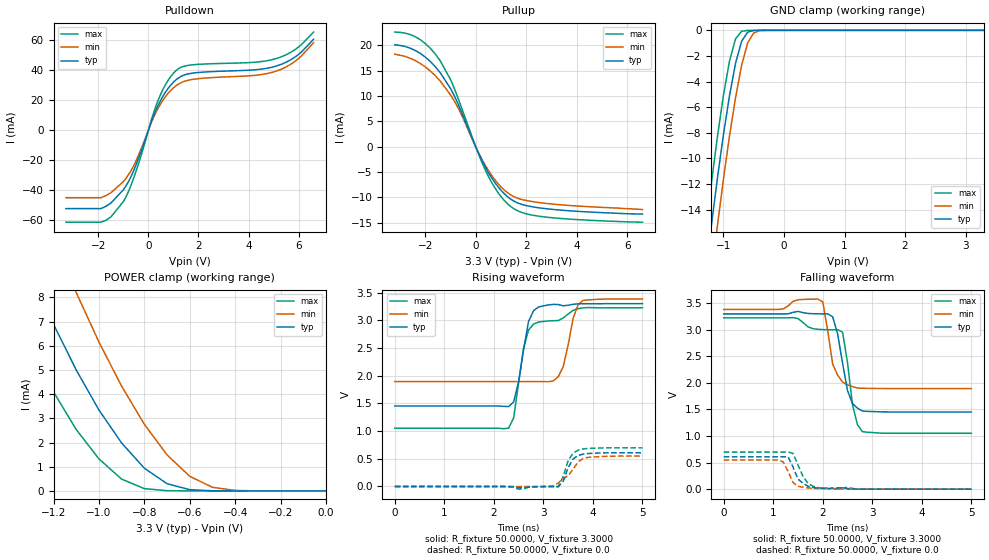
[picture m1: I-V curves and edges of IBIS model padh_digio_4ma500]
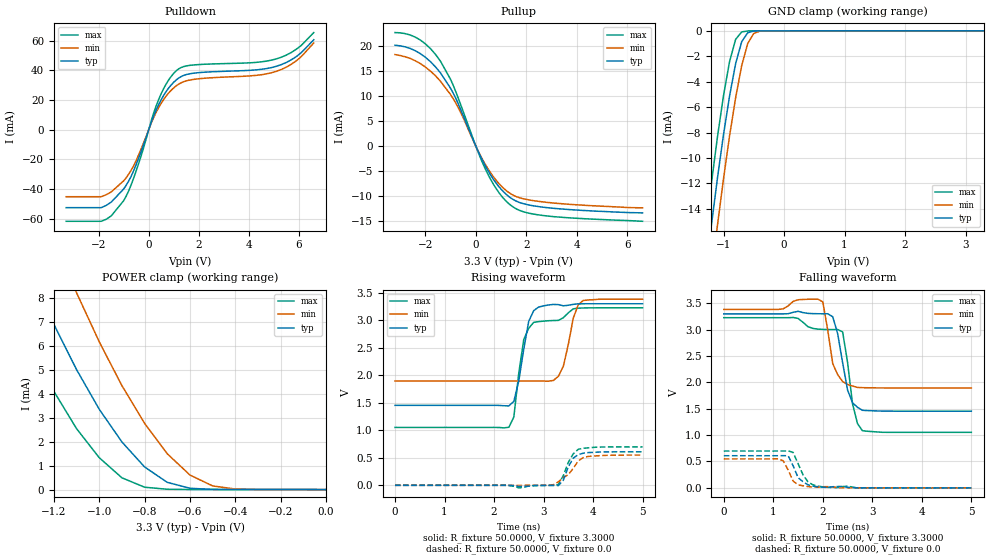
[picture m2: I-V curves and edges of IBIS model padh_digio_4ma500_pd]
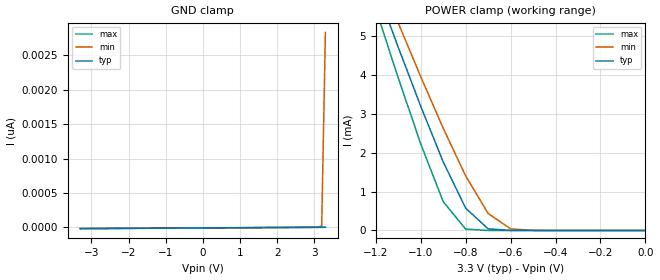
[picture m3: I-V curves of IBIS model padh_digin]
| IBIS file cs4272.ibs created by s2ibis3 verion 1.0
| North Carolina State University, ERL, 2005
[IBIS ver]   3.2
[Comment char]  |_char
[File name]   cs4272.ibs
[File Rev]   1.0B
[Date]   January 26, 2003
[Source]   HSpice Netlist
[Notes]   Rev. 1.0  1/26/2006  28-pin.  Original file.
|   Created by D. DeVries
[Copyright]   (C)opyright 2003 Cirrus Logic, Inc.  All Rights Reserved
[Component]   cs4272
[Manufacturer]  Cirrus Logic, Inc.
|   Component cs4272
[Package]
| variable   typ   min   max
R_pkg   12m   6.8m   16.1m
L_pkg   1.4n   0.713n   2.100n
C_pkg   0.27p   0.180p   0.368p
[Pin]  signal_name   model_name   R_pin   L_pin   C_pin
1   XTO   NC
2   XTI   NC
3   MCLK   padh_digio_mclk_pd
4   LRCK   padh_digio_4ma500
5   SCLK   padh_digio_4ma500
6   SDOUT   padh_digio_4ma500_pd
7   SDIN   padh_digin
8   DGND   GND
9   VD   POWER
10   VL   POWER
11   SCL_CCLK   padh_digin
12   SDA_CDIN   padh_digio_mclk
13   AD0_CSB   padh_digin
14   RSTB   padh_digin
15   VCOM   NC
16   AINA-   NC
17   AINA+   NC
18   AINB+   NC
19   AINB-   NC
20   VA   POWER
21   AGND   GND
22   FILT+   NC
23   AMUTECB   NC
24   AOUTA-   NC
25   AOUTA+   NC
26   AOUTB+   NC
27   AOUTB-   NC
28   BMUTECB   NC
| Models and submodels in the file (5): padh_digio_4ma500 (I/O), padh_digio_4ma500_pd (I/O), padh_digin (Input), padh_digio_mclk (I/O), padh_digio_mclk_pd (I/O)
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|   Model sclk
[Model]  padh_digio_4ma500
Model_type I/O
Polarity   Non-Inverting
Enable   Active-High
Vinl =   0.8000V
Vinh =   2.0000V
C_comp   5.0000pF   5.0000pF   5.0000pF
[Temperature Range]   25.0000   85.0000   -40.0000
[Voltage Range]   3.3000V   3.0000V   3.6000V
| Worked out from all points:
|   slope of the pulldown table from 0 to 0.495 V, typ, clamps not added: 24.7 ohm
|   slope of the pullup table from 0 to 0.495 V, typ, clamps not added: 98.8 ohm
|   GND clamp passes 1 mA (typ) near -0.71 V on its own axis
|   POWER clamp passes 1 mA (typ) near -0.81 V on its own axis
|   rising waveform, R_fixture 50.0000, V_fixture 3.3000: 20-80 % time 211ps typ, 213ps min, 251ps max; typ from 1.45 V to 3.3 V
|   rising waveform, R_fixture 50.0000, V_fixture 0.0: 20-80 % time 183ps typ, 339ps min, 190ps max; typ from 0 V to 0.609 V
|   falling waveform, R_fixture 50.0000, V_fixture 3.3000: 20-80 % time 215ps typ, 197ps min, 199ps max; typ from 3.3 V to 1.45 V
|   falling waveform, R_fixture 50.0000, V_fixture 0.0: 20-80 % time 224ps typ, 180ps min, 225ps max; typ from 0.609 V to 0 V
[Pulldown]
|Voltage   I(typ)   I(min)   I(max)
-3.3V     -52.63mA   -45.34mA   -61.73mA
-1.9V     -52.63mA   -45.34mA   -61.73mA
-1.5V     -48.89mA   -42.01mA   -58.21mA
-1V       -40.01mA   -34.49mA   -47.85mA
-500mV    -23.46mA   -20.77mA   -27.75mA
400mV     16.95mA    14.97mA    20.47mA
800mV     28.15mA    24.8mA     33.6mA
1.2V      34.82mA    30.69mA    41.03mA
1.8V      38.11mA    33.92mA    43.66mA
5.1V      42.72mA    39.33mA    47.72mA
5.9V      49.29mA    46.44mA    54.23mA
6.6V      60.64mA    58.39mA    65.5mA
[Pullup]
|Voltage   I(typ)   I(min)   I(max)
-3.2V     20.09mA    18.25mA    22.61mA
-2.2V     18.43mA    16.44mA    21.14mA
-1.4V     14.58mA    12.93mA    16.92mA
-1V       11.52mA    10.26mA    13.29mA
-700mV    8.48mA     7.707mA    9.604mA
100mV     -1.136mA   -1.073mA   -1.316mA
400mV     -4.167mA   -3.86mA    -4.805mA
900mV     -8mA       -7.381mA   -9.169mA
1.4V      -10.39mA   -9.555mA   -11.86mA
1.9V      -11.49mA   -10.51mA   -13.1mA
2.8V      -12.25mA   -11.2mA    -13.91mA
6.6V      -13.3mA    -12.4mA    -14.9mA
[GND_clamp]
|Voltage   I(typ)   I(min)   I(max)
-3.3V     -106.5mA   -108.9mA   -107mA
-1.3V     -19.19mA   -23.13mA   -15.94mA
-1.2V     -15.28mA   -19.12mA   -11.98mA
-1.1V     -11.57mA   -15.28mA   -8.331mA
-1V       -8.145mA   -11.63mA   -5.085mA
-900mV    -5.12mA    -8.256mA   -2.402mA
-800mV    -2.575mA   -5.266mA   -663.9uA
-700mV    -853.9uA   -2.734mA   -79.03uA
-600mV    -146.2uA   -989.3uA   -4.169uA
-500mV    -12.66uA   -202.1uA   -123.3nA
-400mV    -717.4nA   -22.85uA   -2.49nA
3.3V      69.94pA    479.2nA    62.99pA
[POWER_clamp]
|Voltage   I(typ)   I(min)   I(max)
-3.3V     67.56mA    73.82mA    64.01mA
-1.4V     11.23mA    15.35mA    7.972mA
-1.3V     8.971mA    12.82mA    5.918mA
-1.2V     6.884mA    10.43mA    4.093mA
-1.1V     4.997mA    8.198mA    2.536mA
-1V       3.345mA    6.155mA    1.325mA
-900mV    1.981mA    4.328mA    487.2uA
-800mV    939.3uA    2.755mA    95.74uA
-700mV    299uA      1.489mA    9.484uA
-600mV    51.78uA    603.4uA    549nA
-400mV    325.5nA    21.08uA    380pA
0V        69.94pA    594.9pA    75.26pA
[Ramp]
| variable   typ   min   max
dV/dt_r  0.3655/0.1809n   0.2755/0.2215n   0.4821/0.1500n
dV/dt_f  1.1082/0.1838n   0.8472/0.2207n   1.4124/0.1615n
R_load = 50.0000
[Rising Waveform]
R_fixture= 50.0000
V_fixture= 3.3000
V_fixture_min= 3.6000
V_fixture_max= 3.0000
|time   V(typ)   V(min)   V(max)
0s        1.453V     1.894V     1.052V
2.3ns     1.443V     1.894V     1.055V
2.4ns     1.527V     1.894V     1.24V
2.6ns     2.474V     1.894V     2.495V
2.8ns     3.172V     1.894V     2.93V
3.3ns     3.284V     1.981V     2.994V
3.4ns     3.261V     2.164V     3.042V
3.6ns     3.288V     3.036V     3.179V
3.8ns     3.299V     3.358V     3.224V
5ns       3.3V       3.383V     3.226V
[Rising Waveform]
R_fixture= 50.0000
V_fixture= 0.0
|time   V(typ)   V(min)   V(max)
0s        0V         0V         0V
2.5ns     -22.51mV   -395.7nV   -48.21mV
3.1ns     -834.9uV   -351.5uV   -1.044mV
3.3ns     -5.311mV   62.93mV    -51uV
3.4ns     95.9mV     145mV      180.6mV
3.5ns     340.2mV    194.3mV    469.4mV
3.6ns     496.9mV    311.4mV    601.5mV
3.7ns     560mV      444.3mV    654.5mV
3.9ns     595mV      525.6mV    687.4mV
5ns       609.2mV    549.2mV    698mV
[Falling Waveform]
R_fixture= 50.0000
V_fixture= 3.3000
V_fixture_min= 3.6000
V_fixture_max= 3.0000
|time   V(typ)   V(min)   V(max)
0s        3.3V       3.383V     3.226V
1.4ns     3.328V     3.536V     3.23V
2ns       3.3V       3.526V     3.004V
2.2ns     3.244V     2.356V     3V
2.4ns     2.373V     2.016V     2.957V
2.5ns     1.853V     1.961V     2.377V
2.6ns     1.613V     1.931V     1.59V
2.7ns     1.526V     1.904V     1.215V
2.8ns     1.47V      1.899V     1.083V
5ns       1.453V     1.894V     1.052V
[Falling Waveform]
R_fixture= 50.0000
V_fixture= 0.0
|time   V(typ)   V(min)   V(max)
0s        609.2mV    549.2mV    698.1mV
1.1ns     609.1mV    551.3mV    698mV
1.2ns     611.3mV    513.5mV    698mV
1.3ns     608.2mV    333.8mV    700.8mV
1.4ns     416.1mV    124.5mV    671.6mV
1.5ns     189.1mV    54.47mV    455.7mV
1.6ns     111.8mV    37.6mV     242.9mV
1.7ns     55.27mV    23.59mV    110.2mV
1.9ns     19.35mV    11.16mV    31.28mV
5ns       4.575uV    -1.362uV   5.281uV
|   Model sclk
[Model]  padh_digio_4ma500_pd
Model_type I/O
Polarity   Non-Inverting
Enable   Active-High
Vinl =   0.8000V
Vinh =   2.0000V
C_comp   5.0000pF   5.0000pF   5.0000pF
[Temperature Range]   25.0000   85.0000   -40.0000
[Voltage Range]   3.3000V   3.0000V   3.6000V
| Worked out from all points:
|   slope of the pulldown table from 0 to 0.495 V, typ, clamps not added: 24.7 ohm
|   slope of the pullup table from 0 to 0.495 V, typ, clamps not added: 98.8 ohm
|   GND clamp passes 1 mA (typ) near -0.71 V on its own axis
|   POWER clamp passes 1 mA (typ) near -0.81 V on its own axis
|   rising waveform, R_fixture 50.0000, V_fixture 3.3000: 20-80 % time 210ps typ, 213ps min, 239ps max; typ from 1.45 V to 3.3 V
|   rising waveform, R_fixture 50.0000, V_fixture 0.0: 20-80 % time 185ps typ, 340ps min, 214ps max; typ from 0 V to 0.609 V
|   falling waveform, R_fixture 50.0000, V_fixture 3.3000: 20-80 % time 215ps typ, 197ps min, 200ps max; typ from 3.3 V to 1.45 V
|   falling waveform, R_fixture 50.0000, V_fixture 0.0: 20-80 % time 228ps typ, 184ps min, 227ps max; typ from 0.609 V to 0 V
[Pulldown]
|Voltage   I(typ)   I(min)   I(max)
-3.3V     -52.63mA   -45.25mA   -61.83mA
-1.9V     -52.63mA   -45.25mA   -61.83mA
-1.5V     -48.89mA   -42.02mA   -58.21mA
-1V       -40.01mA   -34.5mA    -47.86mA
-500mV    -23.46mA   -20.77mA   -27.75mA
400mV     16.95mA    14.97mA    20.47mA
800mV     28.15mA    24.81mA    33.6mA
1.2V      34.82mA    30.7mA     41.03mA
1.8V      38.11mA    33.92mA    43.66mA
5.1V      42.73mA    39.33mA    47.73mA
5.9V      49.29mA    46.44mA    54.23mA
6.6V      60.64mA    58.49mA    65.5mA
[Pullup]
|Voltage   I(typ)   I(min)   I(max)
-3.2V     20.1mA     18.24mA    22.62mA
-2.2V     18.43mA    16.45mA    21.14mA
-1.4V     14.59mA    12.93mA    16.91mA
-1V       11.51mA    10.26mA    13.29mA
-700mV    8.481mA    7.707mA    9.603mA
100mV     -1.136mA   -1.074mA   -1.315mA
400mV     -4.166mA   -3.86mA    -4.804mA
900mV     -8mA       -7.381mA   -9.169mA
1.4V      -10.39mA   -9.555mA   -11.85mA
1.9V      -11.49mA   -10.51mA   -13.1mA
2.7V      -12.19mA   -11.14mA   -13.85mA
6.6V      -13.3mA    -12.3mA    -14.98mA
[GND_clamp]
|Voltage   I(typ)   I(min)   I(max)
-3.3V     -106.5mA   -108.9mA   -107mA
-1.3V     -19.2mA    -23.13mA   -15.94mA
-1.2V     -15.29mA   -19.13mA   -11.99mA
-1.1V     -11.57mA   -15.29mA   -8.336mA
-1V       -8.148mA   -11.63mA   -5.089mA
-900mV    -5.124mA   -8.259mA   -2.406mA
-800mV    -2.578mA   -5.268mA   -667.5uA
-700mV    -856.5uA   -2.737mA   -82.16uA
-600mV    -148.4uA   -991.2uA   -6.83uA
-500mV    -14.48uA   -203.7uA   -2.318uA
-400mV    -2.151uA   -24.12uA   -1.738uA
3.3V      3.357uA    3.23uA     4.351uA
[POWER_clamp]
|Voltage   I(typ)   I(min)   I(max)
-3.3V     67.56mA    73.83mA    64.01mA
-1.4V     11.23mA    15.35mA    7.976mA
-1.3V     8.974mA    12.82mA    5.923mA
-1.2V     6.887mA    10.43mA    4.097mA
-1.1V     5.001mA    8.201mA    2.54mA
-1V       3.348mA    6.158mA    1.33mA
-900mV    1.985mA    4.33mA     491.5uA
-800mV    942.6uA    2.758mA    100.1uA
-700mV    302.3uA    1.492mA    13.84uA
-600mV    55.15uA    606.1uA    4.906uA
-400mV    3.685uA    23.83uA    4.356uA
0V        0A         0A         0A
[Ramp]
| variable   typ   min   max
dV/dt_r  0.3655/0.1834n   0.2758/0.2233n   0.4820/0.1603n
dV/dt_f  1.1076/0.1838n   0.8466/0.2206n   1.4118/0.1672n
R_load = 50.0000
[Rising Waveform]
R_fixture= 50.0000
V_fixture= 3.3000
V_fixture_min= 3.6000
V_fixture_max= 3.0000
|time   V(typ)   V(min)   V(max)
0s        1.453V     1.894V     1.052V
2.3ns     1.443V     1.894V     1.055V
2.4ns     1.526V     1.894V     1.24V
2.6ns     2.472V     1.894V     2.647V
2.8ns     3.172V     1.894V     2.961V
3.3ns     3.284V     1.981V     2.997V
3.4ns     3.261V     2.164V     3.046V
3.6ns     3.288V     3.036V     3.207V
3.8ns     3.299V     3.358V     3.223V
5ns       3.299V     3.383V     3.226V
[Rising Waveform]
R_fixture= 50.0000
V_fixture= 0.0
|time   V(typ)   V(min)   V(max)
0s        0V         0V         0V
2.5ns     -22.34mV   -398.9nV   -46.3mV
3.2ns     -968.9uV   11.01mV    -1.245mV
3.3ns     -5.242mV   62.34mV    13.27mV
3.4ns     94.22mV    144.1mV    177.7mV
3.5ns     335.3mV    193.6mV    418.1mV
3.6ns     492.8mV    309.1mV    571.7mV
3.7ns     558mV      441.3mV    654.4mV
3.9ns     594.5mV    524.5mV    680.7mV
5ns       609.1mV    549.1mV    697.9mV
[Falling Waveform]
R_fixture= 50.0000
V_fixture= 3.3000
V_fixture_min= 3.6000
V_fixture_max= 3.0000
|time   V(typ)   V(min)   V(max)
0s        3.299V     3.383V     3.226V
1.4ns     3.328V     3.535V     3.23V
2ns       3.3V       3.526V     3.004V
2.2ns     3.244V     2.356V     3V
2.4ns     2.373V     2.016V     2.957V
2.5ns     1.853V     1.961V     2.377V
2.6ns     1.613V     1.931V     1.593V
2.7ns     1.527V     1.904V     1.218V
2.8ns     1.47V      1.899V     1.083V
5ns       1.453V     1.894V     1.052V
[Falling Waveform]
R_fixture= 50.0000
V_fixture= 0.0
|time   V(typ)   V(min)   V(max)
0s        609.1mV    549.2mV    698mV
1.1ns     609.1mV    551.1mV    697.9mV
1.2ns     611.2mV    514mV      697.9mV
1.3ns     608.2mV    337.3mV    700.6mV
1.4ns     419.1mV    128.9mV    671.9mV
1.5ns     193.9mV    57.16mV    458.8mV
1.6ns     115.5mV    39.26mV    247.6mV
1.7ns     57.45mV    24.56mV    113.6mV
1.9ns     20.07mV    11.54mV    32.33mV
5ns       4.177uV    -2.147uV   6.963uV
|   Model padh_digin
[Model]  padh_digin
Model_type Input
Vinl =   0.8000V
Vinh =   2.0000V
C_comp   5.0000pF   5.0000pF   5.0000pF
[Temperature Range]   25.0000   85.0000   -40.0000
[Voltage Range]   3.3000V   3.0000V   3.6000V
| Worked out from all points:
|   POWER clamp passes 1 mA (typ) near -0.84 V on its own axis
[GND_clamp]
|Voltage   I(typ)   I(min)   I(max)
-3.3V     -19.8pA    -19.07pA   -20.7pA
3V        -900.1fA   -143.9fA   -1.8pA
3.1V      -600.1fA   858.6fA    -1.5pA
3.2V      -300.1fA   19.01pA    -1.2pA
3.3V      0A         2.835nA    -900fA
[POWER_clamp]
|Voltage   I(typ)   I(min)   I(max)
-3.3V     40.87mA    37.86mA    45.08mA
-1.2V     6.274mA    6.747mA    5.694mA
-1.1V     4.711mA    5.337mA    3.925mA
-1V       3.195mA    3.956mA    2.226mA
-900mV    1.764mA    2.629mA    741.3uA
-800mV    572.3uA    1.403mA    34.11uA
-700mV    41.8uA     437uA      266.3nA
-600mV    967.8nA    41.61uA    1.853nA
-500mV    19.92nA    1.821uA    14.35pA
0V        0A         0A         0A
